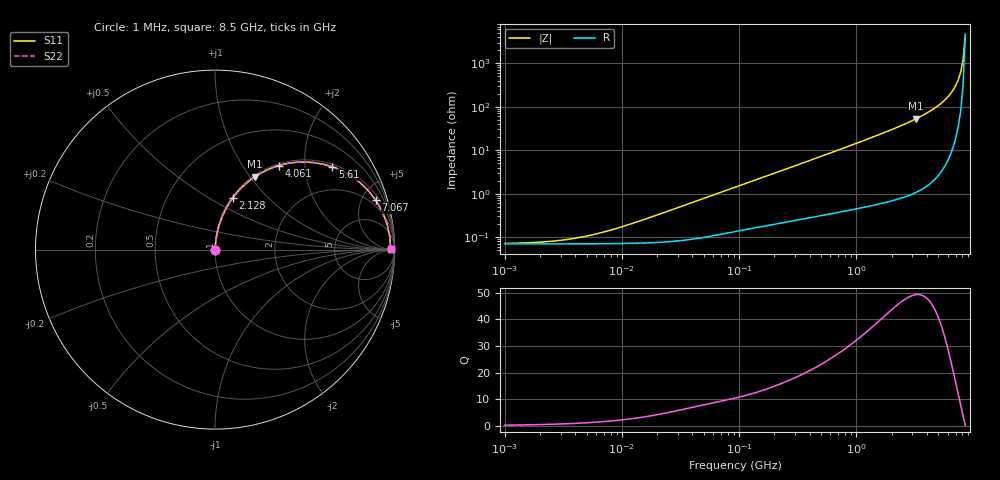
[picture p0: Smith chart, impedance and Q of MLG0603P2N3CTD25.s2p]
! S-Parameter Data Generated by TDK Corporation
! Copyright(C) 2025 TDK Corporation.
! All Rights Reserved.
! TDK P/N: MLG0603P2N3CTD25 (SMD / SMT Inductor (Coil))
! Property: L=2.3nH at 500MHz
! Size(LxWxT): 0.6x0.3x0.3mm
! Model Type: s2p (Touchstone File Format Version 1.0)
! Frequency: DC=Yes Start=1MHz Stop=8500MHz 198points Log-sweep
! Model Generated on Feb. 6, 2025
! Terms and conditions regarding TDK Simulation Models:
! 1)This simulation model is being provided solely for informational
!  purposes. Please refer to the specifications of the products in
!  terms of detailed characteristics of such products.
! 2)In no event shall TDK Corporation of any of its subsidiaries be
!  liable for any loss or damage arising, directly or indirectly,
!  from any information contained in this simulation model, including,
!  but not limited to loss or damages arising from any inaccuracies,
!  omissions or errors in connection with such information.
! 3)Any and all copyrights on this simulation model are owned by
!  TDK Corporation.  Duplication or redistribution of this simulation
!  model without prior written permission from TDK Corporation
!  is prohibited.
! 4)This simulation model is subject to any modification or change
!  without any prior notice.
! 5)Neither TDK Corporation nor any of its subsidiaries shall make any
!  warranty, express or implied, including but not limited to the
!  correctness, implied warranties of merchantability and fitness for
!  a particular purpose with respect to this simulation models.
! 6)The use of this simulation model shall be deemed to have consented
!  to the terms and conditions hereof.
! Port Assignments:
!  1 ---@@@--- 2
! Applicable Conditions:
!  Temperature = 25 degC
!  DC Bias Current = 0 A
!  Small Signal Operation
# Hz S MA R 50
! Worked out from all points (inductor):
!   197 points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, 1 MHz to 8.5 GHz, reference 50 ohm
!   read as one part in series: L = 2.51 nH near 13.89 MHz
!   highest Q = 49.3 at 3.224 GHz (marker M1), where L = 2.61 nH
!   S11 on the Smith chart (normalised r, x): 1 MHz: 1.00, +0.00; 2.128 GHz: 1.01, +0.64; 4.061 GHz: 1.03, +1.47; 5.61 GHz: 1.08, +2.77; 7.067 GHz: 1.40, +6.33; 8.5 GHz: 92, +11
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1000000  0.0007173 12.7  0.9993 -0.0  0.9993 -0.0  0.0007173 12.7
2403882  0.000797 28.5  0.9993 -0.0  0.9993 -0.0  0.000797 28.5
3320851  0.0008762 36.8  0.9993 -0.0  0.9993 -0.0  0.0008762 36.8
4587603  0.00101 45.9  0.9993 -0.0  0.9993 -0.0  0.00101 45.9
8755050  0.001556 62.7  0.9993 -0.1  0.9993 -0.1  0.001556 62.7
2.10461e7  0.003403 76.9  0.9992 -0.2  0.9992 -0.2  0.003403 76.9
9.219544e7  0.01405 83.7  0.9986 -0.8  0.9986 -0.8  0.01405 83.7
4.229561e8  0.06106 83.8  0.9953 -3.5  0.9953 -3.5  0.06106 83.8
9.708683e8  0.1381 80.3  0.9861 -7.9  0.9861 -7.9  0.1381 80.3
1.940355e9  0.2757 72.7  0.9549 -16.0  0.9549 -16.0  0.2757 72.7
2.128028e9  0.3028 71.1  0.9463 -17.6  0.9463 -17.6  0.3028 71.1
2.680511e9  0.3832 66.3  0.9157 -22.5  0.9157 -22.5  0.3832 66.3
3.224109e9  0.4635 61.2  0.8768 -27.6  0.8768 -27.6  0.4635 61.2
4.061159e9  0.5875 52.8  0.797 -36.0  0.797 -36.0  0.5875 52.8
4.884749e9  0.7057 43.8  0.6919 -44.9  0.6919 -44.9  0.7057 43.8
5.610304e9  0.8003 35.2  0.5766 -53.1  0.5766 -53.1  0.8003 35.2
6.44363e9  0.8891 24.9  0.4216 -62.7  0.4216 -62.7  0.8891 24.9
7.066863e9  0.9369 17.1  0.2953 -69.2  0.2953 -69.2  0.9369 17.1
7.400733e9  0.955 13.0  0.2263 -72.1  0.2263 -72.1  0.955 13.0
7.750377e9  0.9684 8.8  0.1543 -73.8  0.1543 -73.8  0.9684 8.8
8.116539e9  0.9765 4.5  0.081 -70.9  0.081 -70.9  0.9765 4.5
8.5e9  0.9789 0.2  0.0213 -6.9  0.0213 -6.9  0.9789 0.2
